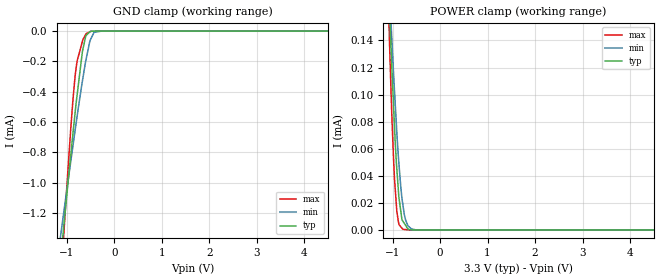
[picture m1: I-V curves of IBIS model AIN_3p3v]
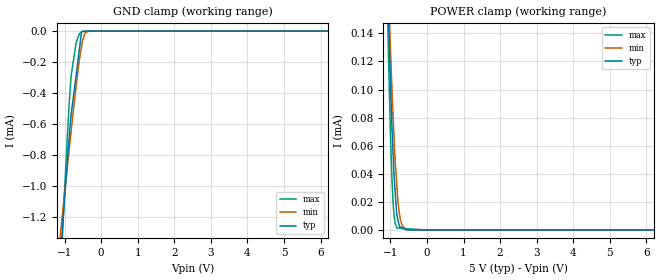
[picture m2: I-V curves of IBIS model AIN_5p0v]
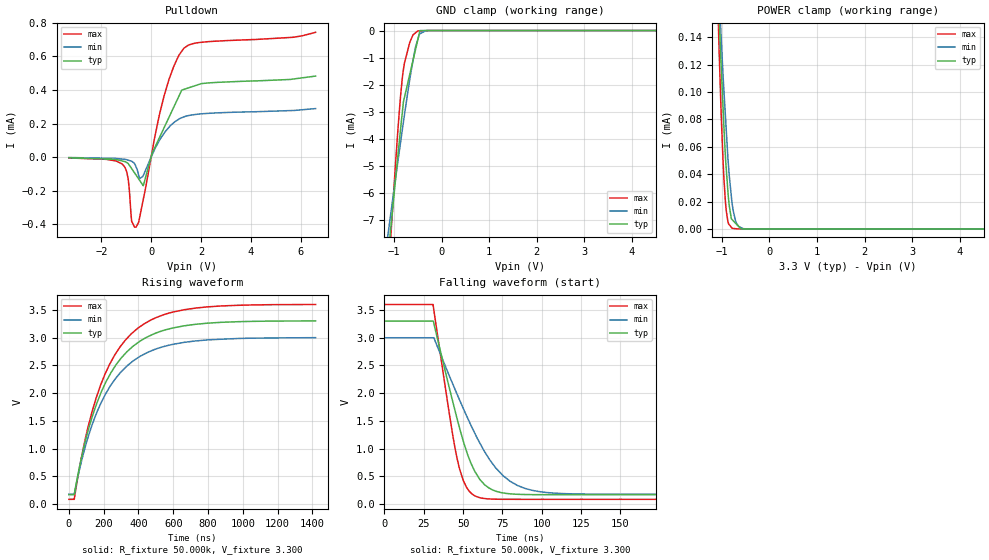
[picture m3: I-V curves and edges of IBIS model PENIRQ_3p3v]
|Texas Instruments Incorporated
|4-wire resistive touch screen controller.
| Marketing part#   Voltage Range   Package-type   #pins
|TSC2003IPW   2.7 to 5.25V   TSSOP   16
|TSC2003IPWG4   2.7 to 5.25V   TSSOP   16
|TSC2003IPWR   2.7 to 5.25V   TSSOP   16
|TSC2003IPWRG4   2.7 to 5.25V   TSSOP   16
[IBIS Ver]   4.0
[File name]   tsc2003ipw.ibs
[File Rev]   1.0
[Date]   02/03/2011
[Source]   Texas Instruments Incorporated.
   Analog-eLab, HPA
   12500 TI Blvd
   Dallas, TX -75243
   For Support e-mail: elab_ibis@list.ti.com
[Notes]   Revision History:
   1.0: 02/03/2011
   - Initial version of the model
   - Initial Model generated from simulations.
   - Model names with a trailing _3p3v contains the model for
   3.3V (3.0V and 3.6V, +/- 10%). Model names with trailing _5p0v
   contains the model for 5V (4.75V and 5.25V, +/- 5%) operation.
   - Model not matched to measurements
   - Please ignore warnings related to non-monotonicity as they
   are from resutls of spice simulations.
[Disclaimer]
 This product is designed as an aid for customers of Texas Instruments.
 No warranties, either expressed or implied, with respect to this third
 party software (if any) or with respect to its fitness for any
 particular purpose is claimed by Texas Instruments or the author. The
 software (if any) is provided solely on an "as is" basis. The entire
 risk as to its quality and performance is with the customer
[Copyright] (C) Copyright 2011 Texas Instruments Incorporated.
   All rights reserved.
|   TSC2003
[Component]   tsc2003ipwr
[Manufacturer] TI
[Package]   | 16 TSSOP  package
| variable   typ   min   max
R_pkg   0.043381   0.0237   0.05823
L_pkg   2.36997nH   2.02293nH   2.90325nH
C_pkg   0.314998pF   0.282pF   0.39476pF
|-------------------------PIN------------------------------------------------
[Pin] signal_name  model_name  R_pin  L_pin C_pin
1   VDD   POWER   0.0237   2.69907nH   0.39476pF
2   X+   TERM   0.05235   2.40523nH   0.30332pF
3   Y+   TERM   0.04146   2.02293nH   0.28442pF
4   X-   TERM   0.04151   2.02647nH   0.282pF
5   Y-   TERM   0.04593   2.18089nH   0.29407pF
6   GND   GND   0.02746   2.06919nH   0.35327pF
7   VBAT1   TERM   0.05823   2.62098nH   0.31095pF
8   VBAT2   TERM   0.04119   2.89055nH   0.35622pF
9   VREF   TERM   0.04155   2.90325nH   0.35922pF
10   PENIRQB PENIRQ   0.04899   2.29328nH   0.29429pF
11   SDA   SDA   0.0469   2.21566nH   0.29234pF
12   SCL   SCL   0.04431   2.12299nH   0.28734pF
13   A1   AIN   0.0442   2.11757nH   0.28675pF
14   A0   AIN   0.04696   2.21273nH   0.2921pF
15   IN2   TERM   0.05191   2.38903nH   0.29903pF
16   IN1   TERM   0.03744   2.74971nH   0.34989pF
[Model Selector] AIN
AIN_3p3v   3.3V Address input
AIN_5p0v   3.3V Address input
[Model Selector] PENIRQ
PENIRQ_3p3v   3.3V Pen interrupt output
PENIRQ_5p0v   5.0V Pen interrupt output
[Model Selector] SCL
SCL_3p3v   3.3V SCL I/O
SCL_5p0v   5.0V SCL I/O
[Model Selector] SDA
SDA_3p3v   3.3V SDA I/O
SDA_5p0v   5.0V SDA I/O
|   TERM Model
[Model] TERM
Model_type Terminator
C_comp   0   0   0
| variable   typ   min   max
[Voltage Range]   3.3V   2.7V   5.25V
[POWER Clamp Reference]  3.3V   2.7V   5.25V
[GND Clamp Reference]   0.0V   0.0V   0.0V
|Operating Temperature
[Temperature Range]   27   85   -40
| Models and submodels in the file (9): AIN_3p3v (Input), AIN_5p0v (Input), PENIRQ_3p3v (Open_drain), PENIRQ_5p0v (Open_drain), SCL_3p3v (I/O_open_drain), SCL_5p0v (I/O_open_drain), SDA_3p3v (I/O_open_drain), SDA_5p0v (I/O_open_drain), TERM (Terminator)
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|   AIN_3p3v
[Model]   AIN_3p3v
Model_type   Input
Vinl = 0.99
Vinh = 2.31
|   typ   min   max
C_comp   1.850pF   1.839pF   1.863pF
[Voltage Range]   3.3   3   3.6
[Temperature Range]   27   85   -40
[Power Clamp Reference]   3.3   3   3.6
[GND Clamp Reference]   0   0   0
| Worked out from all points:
|   GND clamp passes 1 mA (typ) near -0.97 V on its own axis
|   POWER clamp passes 1 mA (typ) near -1.82 V on its own axis
[GND Clamp]
|   Voltage   I(typ)   I(min)   I(max)
-3.3V     -8.902mA   -6.56mA    -13.33mA
-1.157V   -1.602mA   -1.418mA   -1.828mA
-1.058V   -1.278mA   -1.188mA   -1.327mA
-909.5mV  -802.4uA   -849.2uA   -623.4uA
-812.7mV  -508.4uA   -632.4uA   -269.5uA
-782mV    -424.6uA   -565.2uA   -199.2uA
-669mV    -134.1uA   -329.3uA   -68.18uA
-595.8mV  -29.44uA   -192uA     -19.58uA
-499.1mV  -1.584uA   -56.22uA   -2.427uA
-424.1mV  -161.2nA   -8.151uA   -967.8nA
-264.1mV  -24.75nA   -66.25nA   0A
6.6V      0A         0A         0A
[POWER Clamp]
|   Voltage   I(typ)   I(min)   I(max)
-3.3V     2.806mA    2.316mA    3.762mA
-1.157V   254.3uA    255.7uA    259.7uA
-1.066V   164.4uA    181.5uA    141.7uA
-1.058V   158.1uA    175.8uA    132.7uA
-1.023V   126.8uA    147.3uA    93.87uA
-958.5mV  76.57uA    102.8uA    38uA
-909.5mV  45.33uA    72.47uA    13.9uA
-867.1mV  24.65uA    49.85uA    4.791uA
-782mV    6.512uA    18.73uA    478.1nA
-676.6mV  803.6nA    3.119uA    73.93nA
-509.9mV  4.581nA    60.72nA    0A
6.6V      0A         0A         0A
|   AIN_5p0v
[Model]   AIN_5p0v
Model_type   Input
Vinl = 1.5
Vinh = 3.5
|   typ   min   max
C_comp   1.849pF   1.838pF   1.862pF
[Voltage Range]   5   4.75   5.25
[Temperature Range]   27   85   -40
[Power Clamp Reference]   5   4.75   5.25
[GND Clamp Reference]   0   0   0
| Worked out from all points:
|   GND clamp passes 1 mA (typ) near -0.97 V on its own axis
[GND Clamp]
|   Voltage   I(typ)   I(min)   I(max)
-5V       -14.77mA   -10.7mA    -22.57mA
-1.126V   -1.5mA     -1.344mA   -1.667mA
-1.051V   -1.256mA   -1.171mA   -1.29mA
-902.6mV  -780.7uA   -832.8uA   -593.6uA
-820.1mV  -543uA     -648.3uA   -290.6uA
-682mV    -283.1uA   -355uA     -74.64uA
-601.3mV  -131.3uA   -201.7uA   -20.98uA
-534.1mV  -4.92uA    -99.24uA   -6.678uA
-511.6mV  -2.058uA   -66.65uA   -2.751uA
-434.4mV  -643.6nA   -11.03uA   -2.038uA
-341.5mV  -232.3nA   -473.4nA   -1.18uA
10V       0A         0A         0A
[POWER Clamp]
|   Voltage   I(typ)   I(min)   I(max)
-5V       4.92mA     4.029mA    6.652mA
-1.126V   224.8uA    228.9uA    217.3uA
-1.051V   153.8uA    169.5uA    124.1uA
-1.015V   119.3uA    141.1uA    86.04uA
-968.6mV  82.96uA    108.9uA    45.21uA
-919.1mV  50.9uA     78.12uA    17.5uA
-869.6mV  27.76uA    50.79uA    5.167uA
-820.1mV  11.11uA    31.26uA    1.349uA
-790.6mV  6.902uA    20.16uA    1.3uA
-723.5mV  1.957uA    7.103uA    1.187uA
-589.4mV  571.5nA    445.5nA    961.7nA
10V       0A         0A         0A
|   PENIRQ_3p3v
[Model]   PENIRQ_3p3v
Model_type   Open_drain
Polarity   Non-Inverting
Enable   Active-High
Vmeas = 1.65
Vref = 1.65
Cref = 1pF
Rref = 50
|   typ   min   max
C_comp   1.402pF   1.214pF   1.883pF
[Voltage Range]   3.3   3   3.6
[Temperature Range]   27   85   -40
[Pullup Reference]   3.3   3   3.6
[Pulldown Reference]   0   0   0
[Power Clamp Reference]   3.3   3   3.6
[GND Clamp Reference]   0   0   0
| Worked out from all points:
|   slope of the pulldown table from 0 to 0.495 V, typ, clamps not added: 2.98 kohm
|   GND clamp passes 1 mA (typ) near -0.59 V on its own axis
|   POWER clamp passes 1 mA (typ) near -1.83 V on its own axis
|   falling waveform, R_fixture 50.000k, V_fixture 3.300: 20-80 % time 17.9ns typ, 28.9ns min, 11.9ns max; typ from 3.3 V to 0.167 V
|   rising waveform, R_fixture 50.000k, V_fixture 3.300: 20-80 % time 243ns typ, 246ns min, 241ns max; typ from 0.167 V to 3.3 V
[Pulldown]
|   Voltage   I(typ)   I(min)   I(max)
-3.3V     -3.956uA   -2.611uA   -5.18uA
-1.157V   -23.19uA   -11.69uA   -41.37uA
-925.9mV  -37.72uA   -18.03uA   -126.2uA
-782.9mV  -67.83uA   -24.65uA   -380.9uA
-600.6mV  -107.8uA   -59.61uA   -417.3uA
-465.4mV  -137.4uA   -128.9uA   -363.2uA
-313mV    -170.8uA   -110uA     -251.5uA
41.72mV   23.1uA     13uA       33.52uA
520.6mV   174.7uA    141.6uA    364.4uA
916.6mV   300uA      205.7uA    543.4uA
1.313V    403.2uA    239.3uA    648.6uA
6.6V      482.7uA    289uA      743.5uA
[GND Clamp]
|   Voltage   I(typ)   I(min)   I(max)
-3.3V     -50.1mA    -36.94mA   -74.62mA
-1.157V   -8.98mA    -7.952mA   -10.2mA
-1.058V   -7.152mA   -6.657mA   -7.404mA
-909.5mV  -4.479mA   -4.74mA    -3.492mA
-860.6mV  -3.632mA   -4.122mA   -2.41mA
-813mV    -2.833mA   -3.53mA    -1.588mA
-782.9mV  -2.494mA   -3.158mA   -1.225mA
-666.4mV  -1.61mA    -1.792mA   -429.6uA
-550.9mV  -732.5uA   -634uA     -90.09uA
-499.9mV  -345.2uA   -333.4uA   -15.13uA
-454.8mV  -2.816uA   -120.2uA   -12.61uA
6.6V      0A         0A         0A
[POWER Clamp]
|   Voltage   I(typ)   I(min)   I(max)
-3.3V     2.77mA     2.286mA    3.714mA
-1.157V   251uA      252.4uA    256.3uA
-1.066V   162.3uA    179.1uA    139.8uA
-1.023V   125.2uA    145.4uA    92.65uA
-974.8mV  88.08uA    111.5uA    49.17uA
-925.9mV  53.45uA    82.63uA    19.98uA
-876.9mV  29.06uA    53.83uA    6.146uA
-845.1mV  16.94uA    38.97uA    3.121uA
-782.9mV  6.761uA    18.12uA    469.9nA
-693.5mV  3.465uA    4.175uA    109.5nA
-550.9mV  29.89nA    196.3nA    0A
6.59V     0A         0A         0A
[Ramp]
R_load = 50000
|   typ   min   max
dV/dt_r   1.90697/2.43344e-007   1.69387/2.46233e-007   2.10815/2.40669e-007
dV/dt_f   1.90862/1.78771e-008   1.69465/2.89337e-008   2.1098/1.1914e-008
[Falling Waveform]
R_fixture = 50.000k
V_fixture = 3.300
V_fixture_min = 3.000
V_fixture_max = 3.600
C_fixture = 0.000
|  time   V(typ)   V(min)   V(max)
0s        3.301V     3V         3.6V
30.89ns   3.301V     3V         3.598V
43.27ns   1.864V     2.176V     1.268V
47.89ns   1.357V     1.867V     618.6mV
53.95ns   810.4mV    1.483V     227.9mV
65.11ns   316.1mV    878.6mV    93.28mV
75.6ns    198.3mV    504.9mV    84.34mV
84.82ns   174.3mV    330.4mV    83.72mV
120.3ns   166.9mV    181.9mV    83.63mV
1.418us   166.8mV    175.5mV    83.61mV
[Rising Waveform]
R_fixture = 50.000k
V_fixture = 3.300
V_fixture_min = 3.000
V_fixture_max = 3.600
C_fixture = 0.000
|  time   V(typ)   V(min)   V(max)
0s        166.8mV    175.5mV    83.61mV
30.84ns   167.5mV    176.4mV    84.07mV
95.49ns   1.141V     1.045V     1.189V
133.3ns   1.564V     1.423V     1.665V
184.1ns   2.002V     1.818V     2.157V
270ns     2.505V     2.271V     2.717V
393.3ns   2.901V     2.63V      3.162V
540ns     3.126V     2.834V     3.407V
729ns     3.24V      2.94V      3.533V
1.418us   3.301V     2.999V     3.597V
